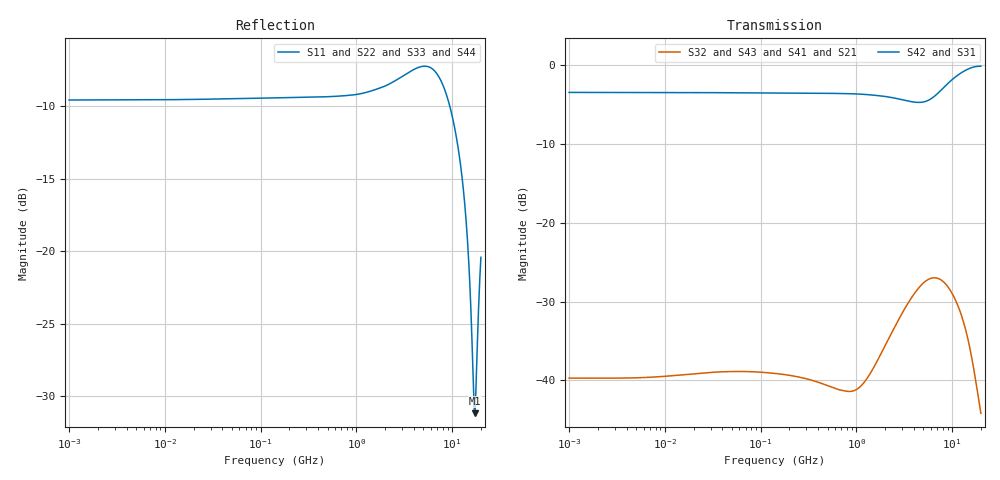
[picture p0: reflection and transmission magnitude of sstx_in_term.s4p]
! Created Mon Mar 13 11:22:51 2017
# hz S ma R 50
! 4 Port Network Data from SP1.SP block
! freq  magS11  angS11  magS12  angS12  magS13  angS13  magS14  angS14
!  magS21  angS21  magS22  angS22  magS23  angS23  magS24  angS24
!  magS31  angS31  magS32  angS32  magS33  angS33  magS34  angS34
!  magS41  angS41  magS42  angS42  magS43  angS43  magS44  angS44
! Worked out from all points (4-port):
!   861 points, 1 MHz to 20 GHz, reference 50 ohm
!   strongest paths, dB at 1 MHz, 11.89 MHz, 141.4 MHz, 1.682 GHz, 20 GHz:
!     S42: -3.5, -3.5, -3.6, -3.9, -0.2
!     S31: -3.5, -3.5, -3.6, -3.9, -0.2
!     S32: -39.7, -39.4, -39.1, -37.4, -44.2
!     S43: -39.7, -39.4, -39.1, -37.4, -44.2
!     S41: -39.7, -39.4, -39.1, -37.4, -44.2
!     S21: -39.7, -39.4, -39.1, -37.4, -44.2
!   lowest |S11| = -31.2 dB at 17.22 GHz (marker M1), VSWR 1.06, Z = 47.4 - j0.458 ohm
!   |S11| at or under -10 dB: 9.469 GHz to end of sweep
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1000000  0.3323 -178.7  0.01035 2.5  0.6678 -0.6  0.01035 2.5
         0.01035 2.5  0.3312 -178.7  0.01035 2.5  0.6689 -0.6
         0.6678 -0.6  0.01035 2.5  0.3323 -178.7  0.01035 2.5
         0.01035 2.5  0.6689 -0.6  0.01035 2.5  0.3312 -178.7
9.240814e8  0.3461 -177.6  0.00858 14.4  0.6544 -1.3  0.00858 14.4
            0.008585 14.3  0.3451 -177.6  0.008585 14.3  0.6554 -1.3
            0.6544 -1.3  0.00858 14.4  0.3461 -177.6  0.00858 14.4
            0.008585 14.3  0.6554 -1.3  0.008585 14.3  0.3451 -177.6
6.178853e9  0.4263 161.0  0.04456 -58.6  0.6128 13.1  0.04456 -58.6
            0.04418 -58.6  0.4225 161.1  0.04418 -58.6  0.6157 12.8
            0.6128 13.1  0.04456 -58.6  0.4263 161.0  0.04456 -58.6
            0.04418 -58.6  0.6157 12.8  0.04418 -58.6  0.4225 161.1
1.218929e10  0.2015 129.8  0.02713 -177.6  0.8848 10.1  0.02713 -177.6
             0.02699 -177.2  0.2012 130.6  0.02699 -177.2  0.8823 10.0
             0.8848 10.1  0.02713 -177.6  0.2015 129.8  0.02713 -177.6
             0.02699 -177.2  0.8823 10.0  0.02699 -177.2  0.2012 130.6
1.44876e10  0.109 126.8  0.01882 144.7  0.9388 5.3  0.01882 144.7
            0.01874 145.1  0.1098 127.8  0.01874 145.1  0.9367 5.3
            0.9388 5.3  0.01882 144.7  0.109 126.8  0.01882 144.7
            0.01874 145.1  0.9367 5.3  0.01874 145.1  0.1098 127.8
1.721926e10  0.02757 -169.9  0.01093 106.2  0.9729 -0.3  0.01093 106.2
             0.0109 106.7  0.02871 -170.5  0.0109 106.7  0.9717 -0.3
             0.9729 -0.3  0.01093 106.2  0.02757 -169.9  0.01093 106.2
             0.0109 106.7  0.9717 -0.3  0.0109 106.7  0.02871 -170.5
2e10  0.09522 -103.8  0.006191 76.8  0.9816 -5.4  0.006191 76.8
      0.006172 77.3  0.09538 -104.3  0.006172 77.3  0.9809 -5.4
      0.9816 -5.4  0.006191 76.8  0.09522 -103.8  0.006191 76.8
      0.006172 77.3  0.9809 -5.4  0.006172 77.3  0.09538 -104.3
